VAR_GLOBAL
	
SMD23K_data: dut_amci_stepper ;

b_relative_move_1_button: BOOL; 
b_absolute_move_1_button: BOOL;
b_jog_cw_1_button: BOOL;
b_jog_ccw_1_button: BOOL; 
b_home_CW_button: BOOL; 
b_reset_errors_button: BOOL;
b_preset_button: BOOL;
b_hold_button: BOOL;
b_program_assembled_move: BOOL;
b_run_blend_move: BOOL; 




END_VAR
